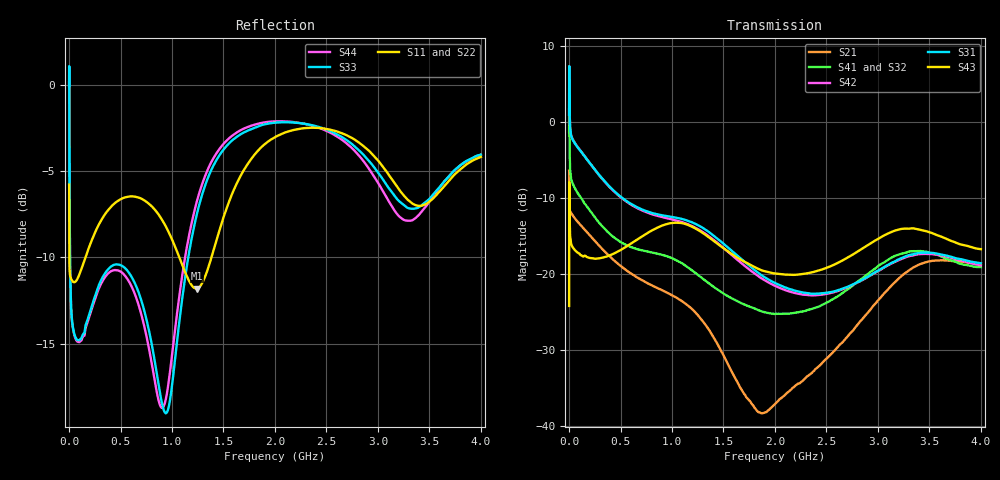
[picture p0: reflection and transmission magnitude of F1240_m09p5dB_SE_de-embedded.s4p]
! Integrated Device Technology
! Corporate Headquarters
! 6024 Silver Creek Valley Road
! San Jose, CA 95138  USA
! Phone:  1-408-284-8200
! Toll Free:  1-800-223-1366
! Webpage:  http://www.idt.com/
! Timing and RF Division
! 515 Groton Road, Suite 102
! Westford, MA 01886-6024
! Device:  F1240
! Description: Dual Intermediate Frequency Digital Variable Gain Amplifier
! Frequency:  10.0 -  500.00 MHz
! Package:  5x5 mm QFN Plastic Package: 32 pin
! Ports:  8 RF, 20 DC
!  Pin  1  = GA3 / Data  Pin 17  = RF OUT_B+
!  Pin  2  = GA4 / CLK  Pin 18  = RF OUT_B-
!  Pin  3  = GA5  Pin 19  = STBY_B
!  Pin  4  = VMODE  Pin 20  = Ground
!  Pin  5  = No Connect  Pin 21  = Ground
!  Pin  6  = GB5  Pin 22  = STB_A
!  Pin  7  = GB4  Pin 23  = RF OUT_A-  = Port 4
!  Pin  8  = GB3  Pin 24  = RF OUT_A+  = Port 3
!  Pin  9  = GB2  Pin 25  = GA0
!  Pin 10  = GB1  Pin 26  = ISET_A
!  Pin 11  = RF IN_B+  Pin 27  = VCC
!  Pin 12  = RF IN_B-  Pin 28  = Ground
!  Pin 13  = Ground  Pin 29  = RF IN_A-  = Port 2
!  Pin 14  = VCC  Pin 30  = RF IN_A+  = Port 1
!  Pin 15  = ISET_B  Pin 31  = GA1
!  Pin 16  = GB0  Pin 32  = GA2 / CSb
! Gain  = +19.5 dB
! State  = 1
! Voltage  = +5.00 V
! Current  = 85.292 mA (one channel only)
! Temperture  =  +25 C
! Test Date  =  2017-10-18
! Board  =  EB4031
! Data:  The device was measured on a custom evaluation board which has
!  individual transmission lines to the RF pins.  Data was collected
!  using a calibrated network analyzer.  The evaluation board was
!  de-embedded using Automatic Fixture Removal.
!  The reference plane is the edge of the package pin.
!  Only Channel A was measured.
!  This data is in single-ended operation.  If your needs are balanced
!  or differential S-parameters then this file needs to be used a
!  linear simulator.
! File Date:  2017-11-10  MJV
! Note:
!  Integrated Device Technology supplies this data as a sample of measured
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# Hz S dB R 100
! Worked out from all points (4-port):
!   410 points, 500 kHz to 4 GHz, reference 100 ohm
!   strongest paths, dB at 500 kHz, 930 MHz, 1.96 GHz, 2.98 GHz, 4 GHz:
!     S43: -24.3, -13.6, -19.9, -15.6, -16.8
!     S31: 0.9, -12.4, -21.0, -19.7, -18.6
!     S42: 0.9, -12.6, -21.3, -19.8, -18.9
!     S41: -1.4, -17.6, -25.3, -19.3, -19.1
!     S32: -1.4, -17.8, -25.0, -19.4, -19.4
!     S21: -6.5, -22.4, -37.7, -23.9, -18.6
!   lowest |S11| = -11.8 dB at 1.24 GHz (marker M1), VSWR 1.69, Z = 60 - j9.88 ohm
!   |S11| at or under -10 dB: 2.967 MHz to 159.5 MHz (156.5 MHz wide, 193 % of centre); 1.071 GHz to 1.383 GHz (311.9 MHz wide, 25.4 % of centre)
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500000  -5.78 -5.6  -6.45 -5.8  -31.83 77.0  -34.08 76.0
        -6.46 -5.8  -5.78 -5.6  -34.03 75.0  -31.84 78.1
        0.92 -111.6  -1.38 -113.5  -0.07 -0.2  -24.26 -38.6
        -1.40 -112.3  0.92 -110.5  -24.26 -38.7  -0.08 2.1
3500000  -10.33 -18.7  -11.23 -17.2  -25.26 3.4  -29.64 -10.8
         -11.22 -17.2  -10.33 -18.9  -29.60 -11.1  -25.26 3.6
         3.27 155.1  -1.11 140.9  -4.05 -84.2  -10.32 175.0
         -1.14 141.1  3.27 155.3  -10.33 175.0  -4.09 -84.2
3.7e8  -7.32 -125.0  -17.41 -99.4  -30.15 -80.2  -37.01 -77.7
       -17.42 -99.3  -7.24 -125.8  -37.09 -76.1  -30.33 -80.3
       -8.22 58.6  -14.52 22.9  -10.75 -163.5  -17.79 48.2
       -14.44 22.1  -8.28 57.2  -17.73 47.8  -10.98 -164.2
1.24e9  -11.80 -162.6  -25.41 102.6  -29.84 121.1  -35.28 151.9
        -25.30 102.4  -11.65 -162.0  -35.08 155.6  -31.16 123.9
        -13.54 -134.9  -20.01 148.0  -7.52 -116.5  -14.33 174.7
        -20.06 140.7  -14.06 -136.2  -14.17 174.8  -6.78 -119.1
2.84e9  -3.46 111.9  -26.12 -10.3  -29.74 -135.7  -32.11 -122.1
        -26.12 -10.4  -3.28 112.4  -32.60 -109.7  -31.05 -127.1
        -20.88 -52.5  -20.90 -129.7  -3.93 105.0  -17.48 -79.5
        -20.71 -140.9  -20.92 -49.0  -16.78 -77.4  -4.27 98.3
3.38e9  -6.99 -3.2  -18.91 -114.1  -26.32 106.2  -28.49 121.8
        -18.94 -114.0  -6.71 0.3  -28.76 136.3  -27.84 114.8
        -17.32 -167.4  -17.04 100.1  -7.14 -19.6  -15.32 168.2
        -17.04 85.9  -17.49 -163.4  -14.15 168.0  -7.64 -35.7
4e9  -4.17 -127.4  -18.64 123.5  -27.27 -19.8  -28.31 -5.1
     -18.64 123.5  -3.94 -126.0  -28.91 8.1  -29.02 -9.3
     -18.64 57.3  -19.37 -36.4  -4.05 -133.0  -18.16 61.5
     -19.14 -50.3  -18.92 63.5  -16.79 55.4  -4.05 -142.9
